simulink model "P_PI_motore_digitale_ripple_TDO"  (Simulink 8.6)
settings: Solver=ode45  StartTime=0.0  StopTime=0.7  RelTol=1e-3
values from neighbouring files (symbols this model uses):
  A = [0,1,0,0;-Kel/Jm,-(Del+Dm)/Jm,Kel/Jm,Del/Jm;0,0,0,1;Kel/Jlr,Del/Jlr,-Kel/Jlr,-Del/Jlr]    [labcontaut5.m]
  B = [0;1/Jm;0;0]    [labcontaut5.m]
  Dm = 0.0034    [labcontaut5.m]
  Jm = 1.5e-4    (= 0.00015)    [labcontaut5.m]
  Kpp = 27    [labcontaut5.m]
  Kt = 1.6    [labcontaut5.m]
  Tf = 0.001    [labcontaut5.m]
  Ts = 0.001    [labcontaut5.m]
undefined symbols (not defined in the file or in its folder): denGf, denRd, denRv, DiscIntNeverNeededParam, numGf, numRd, numRv

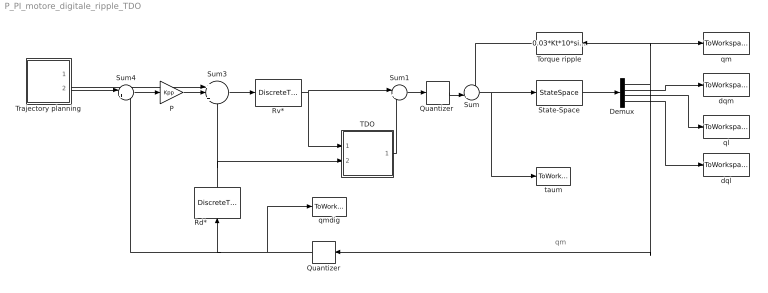
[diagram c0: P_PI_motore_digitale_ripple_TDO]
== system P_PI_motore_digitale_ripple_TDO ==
  note: qm
  Demux : Demux
  P : Gain  Gain=Kpp
  Quantizer : Quantizer  QuantizationInterval=quant_pos
  "Quantizer " : Quantizer  QuantizationInterval=quant_cop
  Rd* : DiscreteTransferFcn  Numerator=numRd  Denominator=denRd  SampleTime=Ts
  Rv* : DiscreteTransferFcn  Numerator=numRv  Denominator=denRv  SampleTime=Ts
  State-Space : StateSpace  A=A  B=B  C=eye(4)  D=zeros(4,1)  X0=[0;0;0;0]
  Sum : Sum  Inputs=++|
  Sum1 : Sum  Inputs=|++
  Sum3 : Sum  Inputs=+|+|-
  Sum4 : Sum  Inputs=|+-
  TDO : Subsystem
  Torque ripple : Fcn  Expr=0.03*Kt*10*sin(3*u)
  Trajectory planning : Subsystem
  dql : ToWorkspace  VariableName=dql  SampleTime=-1
  dqm : ToWorkspace  VariableName=dqm  SampleTime=-1
  ql : ToWorkspace  VariableName=ql  SampleTime=-1
  qm : ToWorkspace  VariableName=qm  SampleTime=-1
  qmdig : ToWorkspace  VariableName=qmdig  SampleTime=-1
  taum : ToWorkspace  VariableName=taum  SampleTime=-1
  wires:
  Sum4/1 -> P/1
  Sum3/1 -> Rv*/1
  P/1 -> Sum3/2
  State-Space/1 -> Demux/1
  Demux/3 -> ql/1
  Demux/4 -> dql/1
  Demux/2 -> dqm/1
  Demux/1 -> Quantizer/1, qm/1, Torque ripple/1
  Rd*/1 -> Sum3/3, TDO/2(dqm)
  Quantizer/1 -> Sum4/2, Rd*/1, qmdig/1
  "Quantizer "/1 -> Sum/2
  Sum/1 -> State-Space/1, taum/1
  Trajectory planning/2(qm°) -> Sum4/1
  Trajectory planning/1(dqm°) -> Sum3/1
  Sum1/1 -> "Quantizer "/1
  Rv*/1 -> Sum1/1, TDO/1(taum)
  Torque ripple/1 -> Sum/1
  TDO/1(taum*) -> Sum1/2

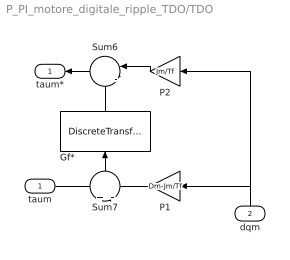
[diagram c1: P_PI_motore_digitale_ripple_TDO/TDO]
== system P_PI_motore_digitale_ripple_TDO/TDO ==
  taum : Inport
  dqm : Inport  Port=2
  Gf* : DiscreteTransferFcn  Numerator=numGf  Denominator=denGf  SampleTime=Ts
  P1 : Gain  Gain=Dm-Jm/Tf
  P2 : Gain  Gain=Jm/Tf
  Sum6 : Sum  Inputs=||-|+
  Sum7 : Sum  Inputs=+|-
  taum* : Outport
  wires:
  P1/1 -> Sum7/2
  Gf*/1 -> Sum6/2
  P2/1 -> Sum6/1
  Sum7/1 -> Gf*/1
  dqm/1 -> P2/1, P1/1
  taum/1 -> Sum7/1
  Sum6/1 -> taum*/1

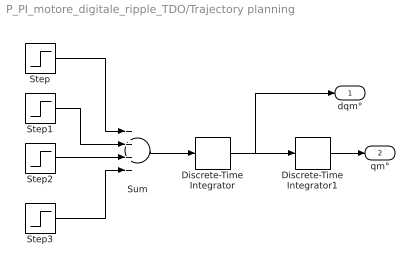
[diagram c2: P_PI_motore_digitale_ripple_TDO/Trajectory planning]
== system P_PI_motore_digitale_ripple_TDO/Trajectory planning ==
  Discrete-Time Integrator : DiscreteIntegrator  IntegratorMethod=Integration: Backward Euler  gainval=1  SampleTime=Ts  ICPrevOutput=DiscIntNeverNeededParam  ICPrevScaledInput=DiscIntNeverNeededParam
  Discrete-Time Integrator1 : DiscreteIntegrator  IntegratorMethod=Integration: Backward Euler  gainval=1  SampleTime=Ts  ICPrevOutput=DiscIntNeverNeededParam  ICPrevScaledInput=DiscIntNeverNeededParam
  Step : Step  Time=0  After=1000  SampleTime=0
  Step1 : Step  Time=0.2  After=-1000  SampleTime=0
  Step2 : Step  Time=0.3  After=-1000  SampleTime=0
  Step3 : Step  Time=0.5  After=1000  SampleTime=0
  Sum : Sum  Inputs=++++
  dqm° : Outport
  qm° : Outport  Port=2
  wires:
  Discrete-Time Integrator/1 -> dqm°/1, Discrete-Time Integrator1/1
  Discrete-Time Integrator1/1 -> qm°/1
  Sum/1 -> Discrete-Time Integrator/1
  Step3/1 -> Sum/4
  Step2/1 -> Sum/3
  Step1/1 -> Sum/2
  Step/1 -> Sum/1
